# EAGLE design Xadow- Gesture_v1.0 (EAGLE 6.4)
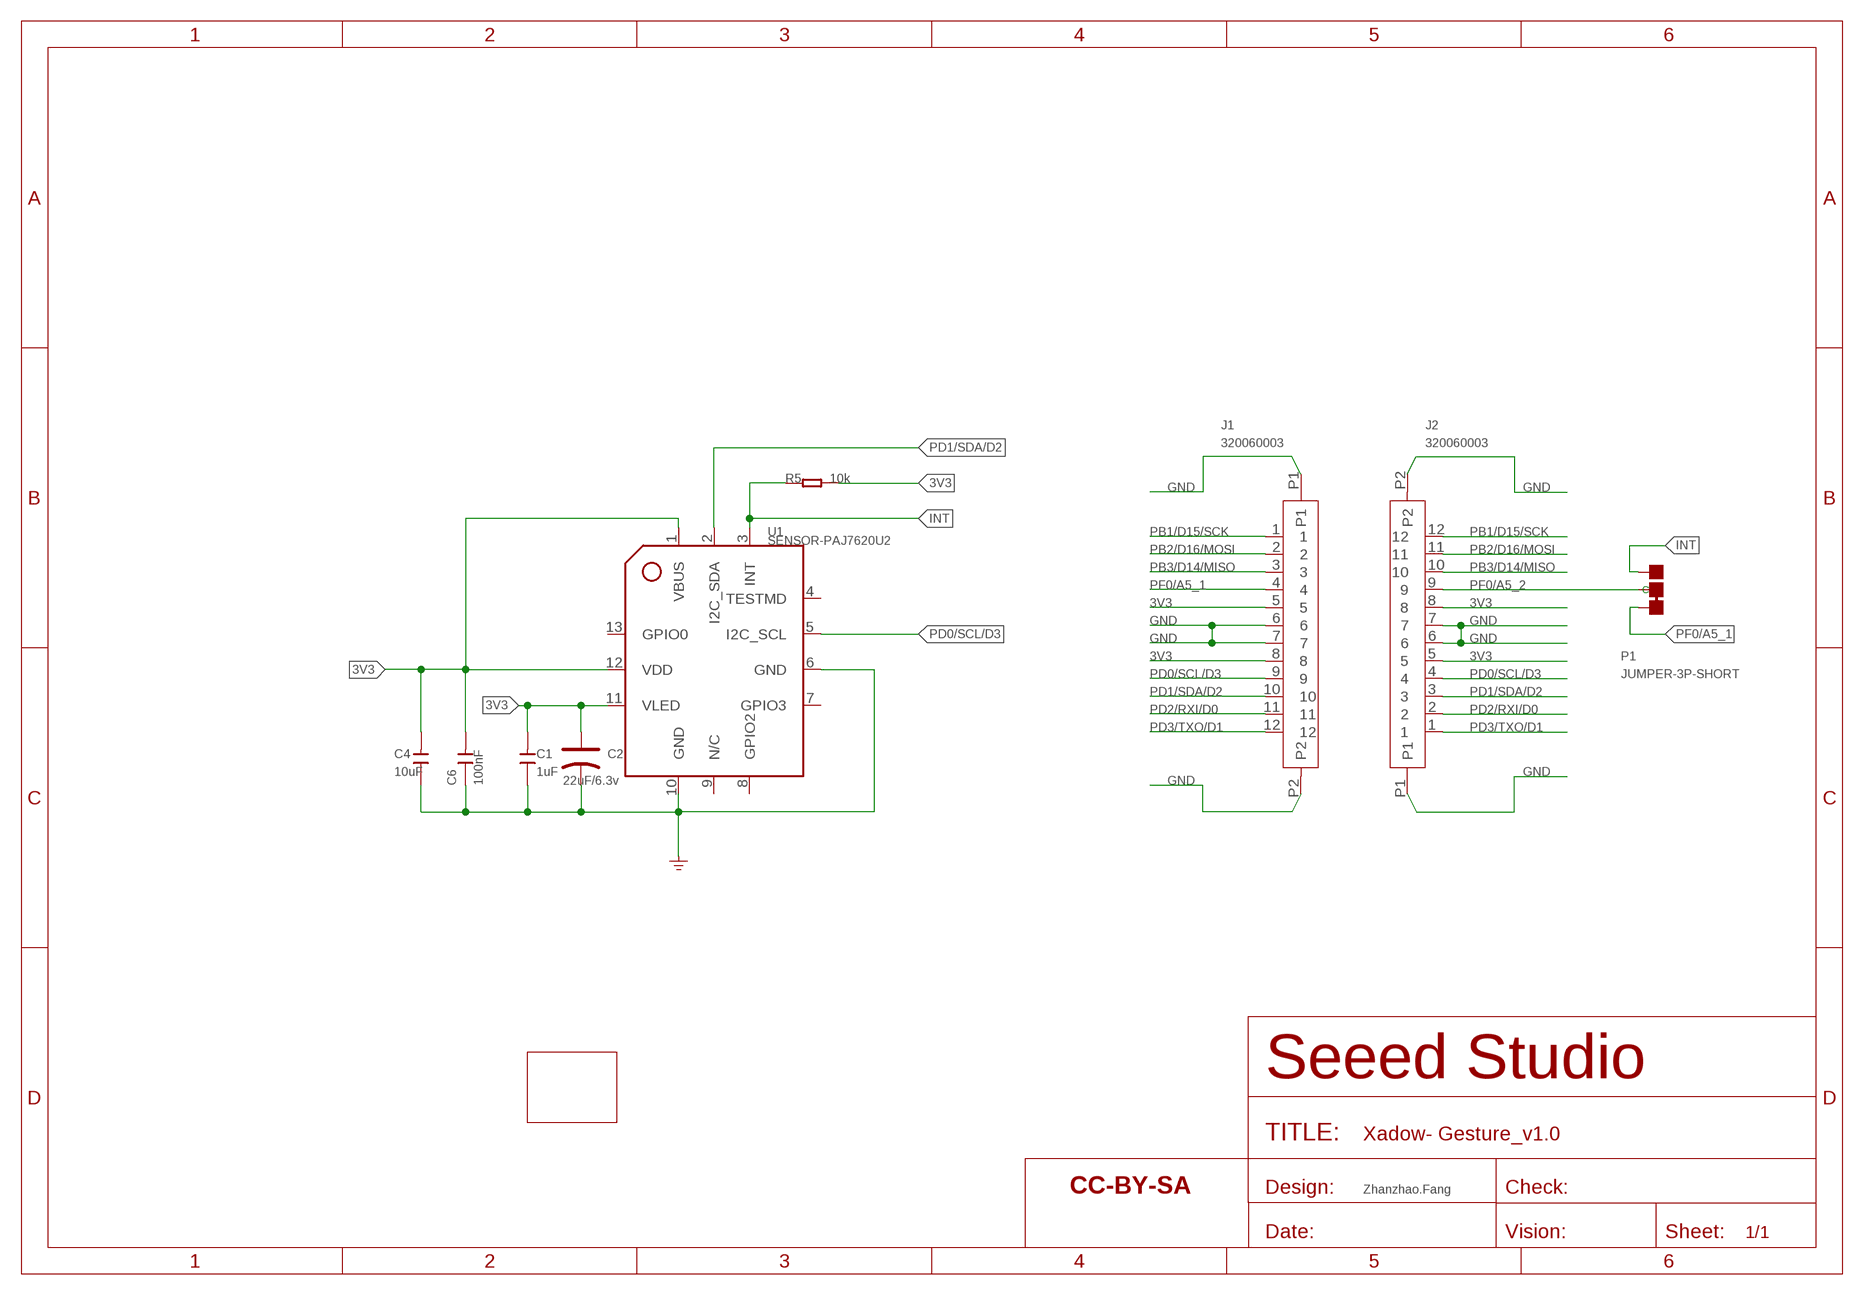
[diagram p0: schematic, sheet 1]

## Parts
C1  1uF  CAP-0603  [C0603]
C2  22uF/6.3v  CAP-POLAR-AVX-A  [AVX-A]
C4  10uF  CAP-0603  [C0603]
C6  100nF  CAP-0603  [C0603]
J1  320060003  FPC-CONNECTOR-12P-FH12-12S-0.5SH  [12P-0.5]
J2  320060003  FPC-CONNECTOR-12P-FH12-12S-0.5SH  [12P-0.5]
P1  JUMPER-3P-SHORT  [3P-SMD_SHORT]
R5  10k  RES-0603  [R0603]
U1  SENSOR-PAJ7620U2  [LGA13-SMD-L5.2*W3*H2MM]
U$4  SEEEDSTUDIO-OPEN-SCH-FRAME  [SEEEDSTUDIO-PCB-FRAME]
U$7  XADOW  [XADOW-DRILL-DIM-25*20MM]

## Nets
3V3: C1.2 C2.+ C4.2 C6.2 J1.5 J1.8 J2.5 J2.8 R5.2 U1.1(VBUS) U1.11(VLED) U1.12(VDD)
GND: C1.1 C2.- C4.1 C6.1 J1.6 J1.7 J1.P1 J1.P2 J2.6 J2.7 J2.P1 J2.P2 U1.6(GND) U1.10(GND) ; supply symbol labelled GND_POWER
INT: P1.00(R) R5.1 U1.3(INT)
PB1/D15/SCK: J1.1 J2.12
PB2/D16/MOSI: J1.2 J2.11
PB3/D14/MISO: J1.3 J2.10
PD0/SCL/D3: J1.9 J2.4 U1.5(I2C_SCL)
PD1/SDA/D2: J1.10 J2.3 U1.2(I2C_SDA)
PD2/RXI/D0: J1.11 J2.2
PD3/TXO/D1: J1.12 J2.1
PF0/A5_1: J1.4 P1.11(L)
PF0/A5_2: J2.9 P1.MM(C)
Unconnected: U1.4(TESTMD) U1.7(GPIO3) U1.8(GPIO2) U1.9(N/C) U1.13(GPIO0)

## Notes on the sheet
- Zhanzhao.Fang

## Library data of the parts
C1 C4 C6 = Discrete-new:CAP: Ceramic Capacitors
C2 = Discrete-new:CAP-POLAR: Electrolytic Capacitors,Tantalum Capacitors and Super Capacitors
J1 J2 = Connector-new:FPC-CONNECTOR-12P: 320060003
P1 = Discrete-new:JUMPER-3P-SHORT
R5 = Discrete-new:RES
U1 = template:SENSOR-PAJ7620U2
U$4 = moudle-new:SEEEDSTUDIO-OPEN-SCH-FRAME
U$7 = moudle-new:XADOW

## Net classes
0 default: width 0.102 mm, drill 0.203 mm, clearance 0.102 mm
3 usbvcc: width 0.203 mm, drill 0.305 mm, clearance 0.203 mm

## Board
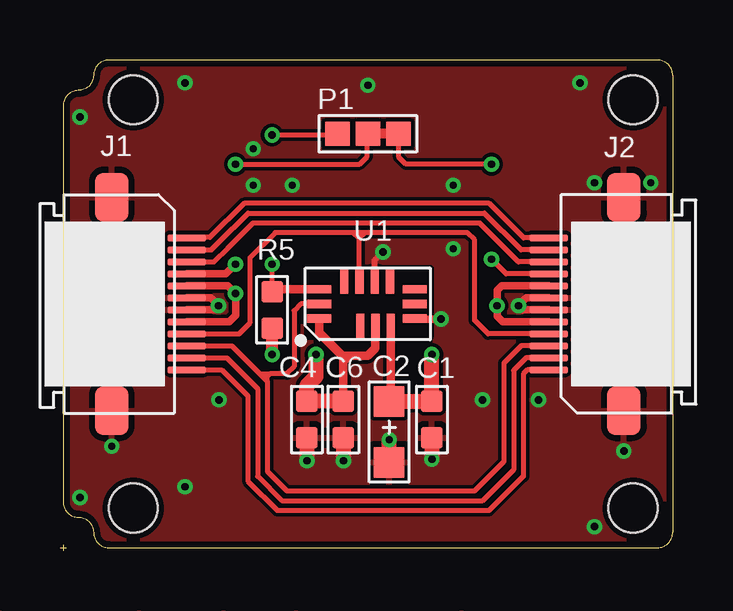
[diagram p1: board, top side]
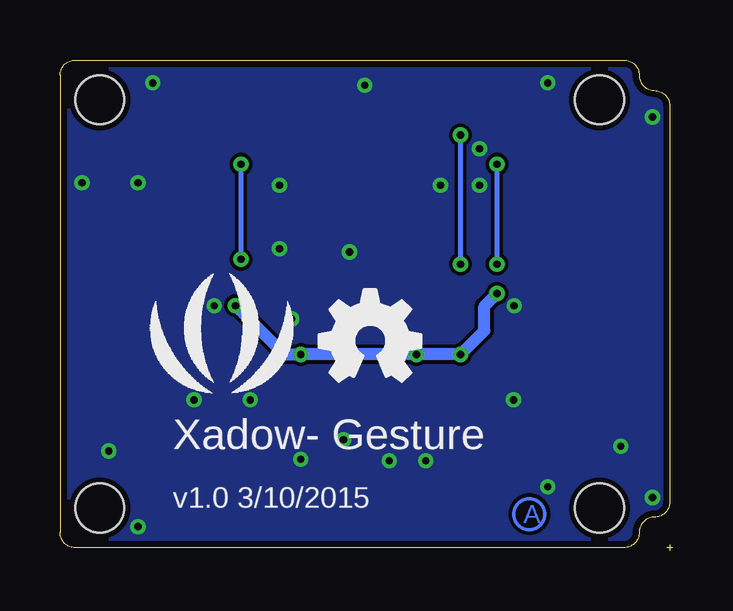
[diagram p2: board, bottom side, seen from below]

Size 25.53 x 20.45 mm. Coordinates in mm from the lower left corner, seen from the top.
Copper layers (1*16): Top 0.035mm / dielectric 1.5mm / Bottom 0.035mm
Design rules "SeeedStudio_2layer_DRU_no_angle_20140221": minimum track width 6mil, minimum drill 12mil, track to track 6mil, track to pad 6mil, pad to pad 6mil, via to via 6mil, smd to smd 0mil, copper to edge 10mil, drill to drill 10mil, minimum pad ring 10mil, minimum via ring 6mil, stop-mask expansion 2mil, vias tented up to drill 25mil, thermal gap 10mil

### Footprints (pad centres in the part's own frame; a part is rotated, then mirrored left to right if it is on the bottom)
C0603 = smd 0.889 x 0.889: 1 0,0.762; 2 0,-0.762
AVX-A = smd 1.27 x 1.27: + -1.27,0; - 1.27,0
12P-0.5 = smd 0.3 x 1.6: 1 -2.75,3.127; 2 -2.25,3.127; 3 -1.75,3.127; 4 -1.25,3.127; 5 -0.75,3.127; 6 -0.25,3.127; 7 0.25,3.127; 8 0.75,3.127; 9 1.25,3.127; 10 1.75,3.127; 11 2.25,3.127; 12 2.75,3.127 | smd 2.032 x 1.397: P1 -4.445,0; P2 4.445,0
3P-SMD_SHORT = smd 1.016 x 1.016: 00 -1.27,0; 11 1.27,0; MM 0,0
R0603 = smd 0.889 x 0.889: 1 0,0.762; 2 0,-0.762
LGA13-SMD-L5.2*W3*H2MM = smd 1 x 0.35: 1 2.02,0.61; 2 2.02,0; 3 2.02,-0.61; 8 -1.96,-0.61; 9 -1.96,0; 10 -1.96,0.61 | smd 0.35 x 1: 4 0.983,-0.92; 5 0.348,-0.92; 6 -0.287,-0.92; 7 -0.922,-0.92; 11 -0.953,0.92; 12 -0.318,0.92; 13 0.318,0.92
XADOW-DRILL-DIM-25*20MM = hole 2.032: -9.779,-8.509; -9.779,8.509; 11.049,8.509; 11.049,-8.509

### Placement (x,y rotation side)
C1  15.49,5.46 180 top
C2  13.72,4.95 270 top
C4  10.29,5.46 180 top
C6  11.81,5.46 180 top
J1  2.16,10.29 270 top
J2  23.49,10.29 90 top
P1  12.83,17.37 0 top
R5  8.84,10.03 0 top
U1  12.83,10.29 180 top
U$4  not placed on the board
U$5  [OSHW_FILLX150_NOTEXT]  14.73,7.06 0 bottom
U$6  [SEEED-SILK-280*268MIL]  18.8,8.28 0 bottom
U$7  12.83,10.29 0 top

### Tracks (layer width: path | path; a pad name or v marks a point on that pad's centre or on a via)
3V3  (via drill 0.3 pad 0.64)
  Top 0.305: J2.8 18.4,11.04 18.21,10.85 v18.21,10.21 18.21,9.78 18.45,9.54 J2.5 | J1.5 7,11.04 v7.32,10.72 7.32,9.8 7.05,9.54 J1.8
  Top 0.356: U1.11 13.78,6.41 C2.+ | U1.12 13.14,8.45 12.83,8.13 12.06,8.13 | U1.1 10.81,9.08 11.76,8.13 11.94,8.13 | 11.94,8.13 12.06,8.13 | C6.2 11.81,7.87 | 11.81,7.87 11.81,8 11.94,8.13 | 12.06,8.13 11.81,7.87
  Top 0.508: v8.84,8.18 R5.2
  Top 0.635: C2.+ C1.2 v15.49,8.18 | C6.2 C4.2 10.29,6.88 10.67,7.26 v10.67,8.18
  Bottom 0.508: v18.21,10.21 16.18,8.18 v15.49,8.18 v10.67,8.18 v8.84,8.18 7.85,9.17 7.85,10.19 v7.32,10.72
GND  (via drill 0.3 pad 0.64)
  Top 0.254: U1.6 13.11,12.1 v13.46,12.45 | 14.81,9.65 U1.10
  Top 0.305: v15.88,9.65 14.81,9.65 | J1.6 6.28,10.54 v6.6,10.21 6.43,10.04 J1.7 | J2.7 19.43,10.54 v19.1,10.21 19.27,10.04 J2.6
  Top 0.635: C4.1 v10.29,3.75 | C6.1 v11.81,3.75 | C2.- v13.72,4.62 | C1.1 v15.49,3.81
  other vias: 5.21,19.49 21.67,19.49 12.83,19.39 16.38,15.23 9.68,15.23 8.05,15.23 5.21,2.67 22.28,1 19.94,6.29 17.6,6.29 16.38,12.59 6.63,6.29 2.16,4.36 23.49,4.15 24.61,15.33 22.28,15.33 8.05,16.75 0.84,18.07 0.84,2.22
  pour Top (rank 6): -1.5,21.77 26.54,21.77 26.54,-0.79 -1.5,-0.79
  pour Bottom (rank 6): -1.5,22.17 26.54,22.17 26.54,-0.38 -1.5,-0.38
INT  (via drill 0.3 pad 0.64)
  Top 0.203: R5.1 v8.84,11.94 | v8.84,17.32 11.51,17.32
  Top 0.356: U1.3 8.74,10.9 R5.1 | 11.51,17.32 P1.00
  Bottom 0.203: v8.84,11.94 v8.84,17.32
N$1
  cutout Top (rank 6): 10.29,11.81 15.47,11.81 15.47,8.86 10.29,8.86
PB1/D15/SCK
  Top 0.203: J2.12 19.32,13.04 17.88,14.48 7.67,14.48 6.25,13.06 5.3,13.06 J1.1
PB2/D16/MOSI
  Top 0.203: J2.11 19.21,12.54 17.68,14.07 7.84,14.07 6.6,12.83 6.31,12.54 J1.2
PB3/D14/MISO
  Top 0.203: J2.10 19.1,12.04 17.48,13.67 8.04,13.67 7.01,12.63 6.42,12.04 J1.3
PD0/SCL/D3
  Top 0.203: 12.19,13.26 8.96,13.26 7.92,12.22 7.92,9.5 7.46,9.04 J1.9 | 12.7,13.26 16.97,13.26 17.27,12.95 17.27,9.6 17.84,9.04 J2.4 | 12.7,13.26 12.5,13.26 | 12.5,13.26 12.19,13.26 | U1.5 12.48,12.99 | 12.48,13.04 12.48,13.24 12.5,13.26 | 12.48,12.99 12.46,12.99 12.19,13.26 | 12.48,12.99 12.48,13.04 | 12.48,13.04 12.7,13.26
PD1/SDA/D2
  Top 0.203: J2.3 19.21,8.54 18.49,7.82 18.49,3.71 17.27,2.49 9.45,2.49 8.64,3.3 8.64,7.06 | J1.10 7.16,8.54 8.33,7.37 | 8.33,7.37 8.74,7.37 | 8.64,7.06 8.33,7.37 | 8.64,7.06 8.64,7.26 8.74,7.37 | U1.2 10.03,10.29 9.75,10.01 9.75,7.67 9.45,7.37 8.74,7.37
PD2/RXI/D0
  Top 0.203: J2.2 19.42,8.04 18.9,7.52 18.9,3.37 17.61,2.08 9.25,2.08 8.23,3.1 8.23,6.76 6.95,8.04 J1.11
PD3/TXO/D1
  Top 0.203: J2.1 19.48,7.54 19.3,7.37 19.3,3.1 17.88,1.68 9.04,1.68 7.82,2.9 7.82,6.45 6.74,7.54 J1.12
PF0/A5_1  (via drill 0.3 pad 0.64)
  Top 0.203: v7.32,16.1 12.48,16.1 12.8,16.43 12.8,17.35 12.83,17.37
  Top 0.305: J1.4 6.91,11.54 v7.32,11.94
  Bottom 0.203: v7.32,11.94 v7.32,16.1
PF0/A5_2  (via drill 0.3 pad 0.64)
  Top 0.203: 14.1,17.37 12.65,17.37 12.6,17.32 | 14.1,17.37 13.06,17.37 13.01,17.32 | v17.98,12.15 v17.98,12.14 18.59,11.54 J2.9 | 14.1,17.37 14.12,17.35 14.12,16.39 14.41,16.1 v17.98,16.1
  Bottom 0.203: v17.98,12.14 v17.98,16.1
(copper drawn outside any net)
  shapes: Bottom circle x1

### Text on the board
Bottom: A
bPlace: Xadow- Gesture | v1.0 3/10/2015

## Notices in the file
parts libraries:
moudle-new: This work is licensed under the Creative Commons Attribution 4.0 International License.
To view a copy of this license,visit:
http://creativecommons.org/licenses/by-sa/4.0
moudle-new: CC-BY-SA
